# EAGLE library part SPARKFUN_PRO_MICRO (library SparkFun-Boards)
SparkFun Pro Micro Atmega32U4 compatible footprint. SparkFun Products: 3.3V/8MHz 5V/16MHz
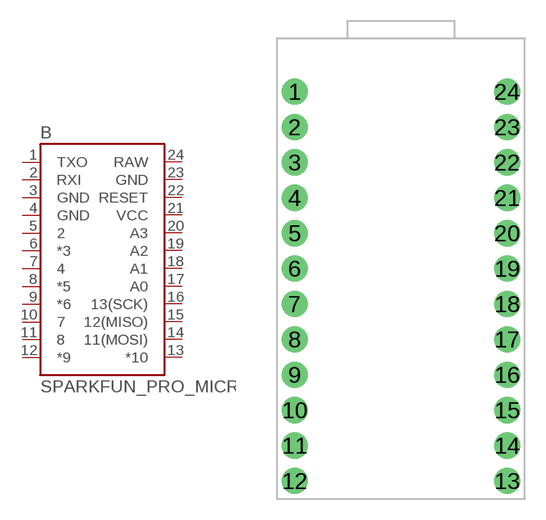
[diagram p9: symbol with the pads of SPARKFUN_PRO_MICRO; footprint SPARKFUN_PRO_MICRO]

Designator prefix B

## SPARKFUN_PRO_MICRO  [SPARKFUN_PRO_MICRO]
1  TXO
2  RXI
3  GND  pwr
4  GND  pwr
5  2
6  *3
7  4
8  *5
9  *6
10  7
11  8
12  *9
13  *10
14  11(MOSI)
15  12(MISO)
16  13(SCK)
17  A0
18  A1
19  A2
20  A3
21  VCC  pwr
22  RESET
23  GND  pwr
24  RAW  pwr

## Footprint SPARKFUN_PRO_MICRO (pad centres in mm)
SparkFun Pro Mico Footprint (with USB connector) Specifications: Pin count: 24 Pin pitch: 0.1" Area:0.7x1.3" Example device(s): SparkFun Pro Micro
drill 1.016 pad 1.88: 1 -7.62,12.7; 2 -7.62,10.16; 3 -7.62,7.62; 4 -7.62,5.08; 5 -7.62,2.54; 6 -7.62,0; 7 -7.62,-2.54; 8 -7.62,-5.08; 9 -7.62,-7.62; 10 -7.62,-10.16; 11 -7.62,-12.7; 12 -7.62,-15.24; 13 7.62,-15.24; 14 7.62,-12.7; 15 7.62,-10.16; 16 7.62,-7.62; 17 7.62,-5.08; 18 7.62,-2.54; 19 7.62,0; 20 7.62,2.54; 21 7.62,5.08; 22 7.62,7.62; 23 7.62,10.16; 24 7.62,12.7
